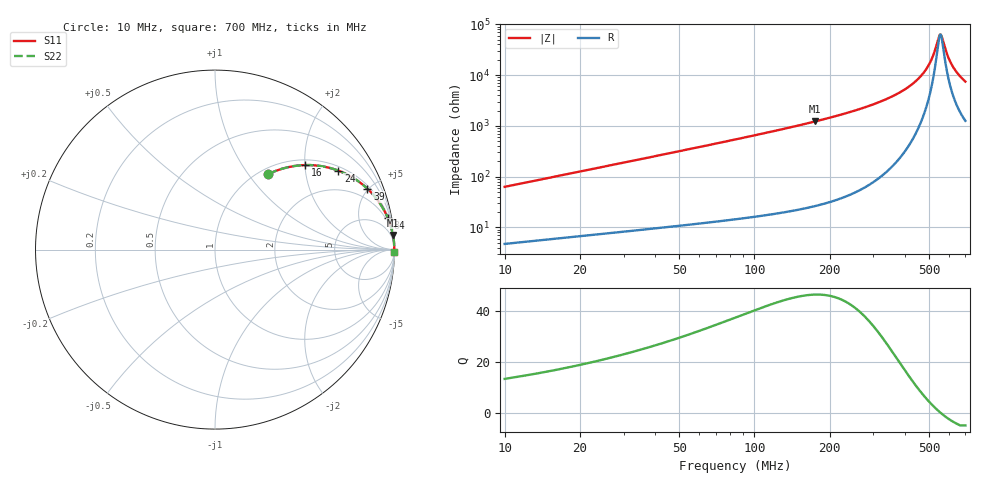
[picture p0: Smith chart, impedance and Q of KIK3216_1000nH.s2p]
!version-2
!date-01.2022
!Series
# MHz S RI R 50
!Freq ReS11 ImS11 ReS21 ImS21 ReS12 ImS12 ReS22 ImS22
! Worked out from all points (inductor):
!   691 points, 10 MHz to 700 MHz, reference 50 ohm
!   read as one part in series: L = 1 uH near 13 MHz
!   highest Q = 46.3 at 175 MHz (marker M1), where L = 1.11 uH
!   self-resonance near 556 MHz
!   S11 on the Smith chart (normalised r, x): 10 MHz: 1.09, +1.26; 16 MHz: 1.12, +2.01; 24 MHz: 1.15, +3.02; 39 MHz: 1.19, +4.93; 84 MHz: 1, +11; 700 MHz: open
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10  0.2981 0.4212  0.7019 -0.4212  0.7019 -0.4212  0.2981 0.4212
16  0.5037 0.471  0.4963 -0.471  0.4963 -0.471  0.5037 0.471
24  0.6874 0.4398  0.3126 -0.4398  0.3126 -0.4398  0.6874 0.4398
31  0.7829 0.3913  0.2171 -0.3913  0.2171 -0.3913  0.7829 0.3913
39  0.8493 0.3391  0.1507 -0.3391  0.1507 -0.3391  0.8493 0.3391
57  0.9222 0.2523  0.0778 -0.2523  0.0778 -0.2523  0.9222 0.2523
84  0.9624 0.1772  0.0376 -0.1772  0.0376 -0.1772  0.9624 0.1772
125  0.983 0.1184  0.017 -0.1184  0.017 -0.1184  0.983 0.1184
175  0.9916 0.0811  0.00839 -0.0811  0.00839 -0.0811  0.9916 0.0811
240  0.9958 0.0536  0.00415 -0.0536  0.00415 -0.0536  0.9958 0.0536
355  0.9982 0.0265  0.0018 -0.0265  0.0018 -0.0265  0.9982 0.0265
421  0.9986 0.0161  0.00144 -0.0161  0.00144 -0.0161  0.9986 0.0161
470  0.9986 0.00965  0.00139 -0.00965  0.00139 -0.00965  0.9986 0.00965
493  0.9986 0.00689  0.00141 -0.00689  0.00141 -0.00689  0.9986 0.00689
512  0.9986 0.00473  0.00145 -0.00473  0.00145 -0.00473  0.9986 0.00473
553  0.9984 0.000334  0.00157 -0.000334  0.00157 -0.000334  0.9984 0.000334
562  0.9984 -0.000585  0.00161 0.000585  0.00161 0.000585  0.9984 -0.000585
585  0.9983 -0.00287  0.00171 0.00287  0.00171 0.00287  0.9983 -0.00287
606  0.9982 -0.00488  0.00182 0.00488  0.00182 0.00488  0.9982 -0.00488
631  0.998 -0.00719  0.00196 0.00719  0.00196 0.00719  0.998 -0.00719
663  0.9978 -0.01  0.00216 0.01  0.00216 0.01  0.9978 -0.01
700  0.9976 -0.0132  0.00243 0.0132  0.00243 0.0132  0.9976 -0.0132
